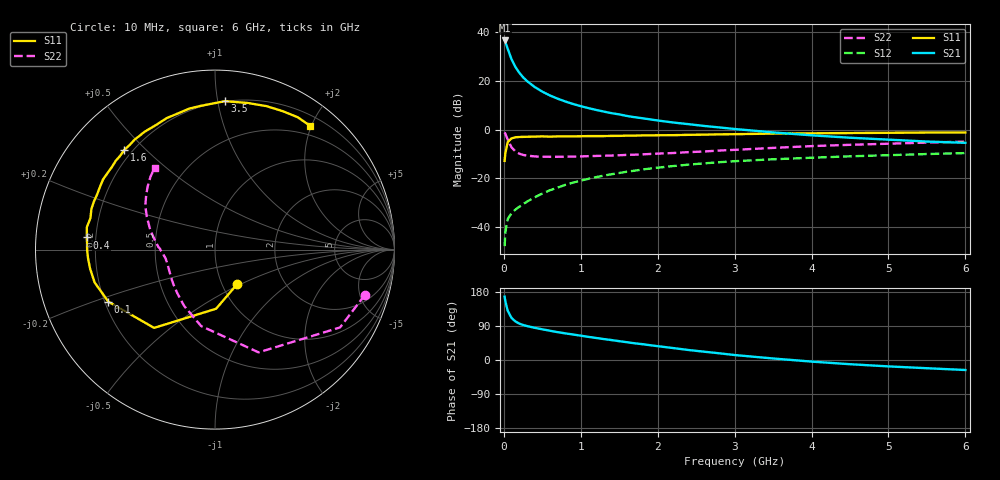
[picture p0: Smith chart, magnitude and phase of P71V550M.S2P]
! SIEMENS Small Signal Semiconductors
! BFP196
! Si NPN RF Bipolar Junction Transistor in SOT143
! VCE = 1.5 V  IC = 50 mA
! Common Emitter S-Parameters:  May  1996
# GHz  S  MA  R  50
!  f  S11  S21  S12  S22
! GHz  MAG  ANG  MAG  ANG  MAG  ANG  MAG  ANG
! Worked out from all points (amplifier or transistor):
!   36 points, 10 MHz to 6 GHz, reference 50 ohm
!   highest |S21| = 36.5 dB at 10 MHz (marker M1)
!   |S21| within 3 dB of that: start of sweep to 45.71 MHz
!   unconditionally stable (mu >= 1): 402.8 MHz to 4.816 GHz
!   at 250 MHz: K = 0.87, MSG = 26.0 dB, |S12| = -30.5 dB
!   at 1.4 GHz: K = 1.09, MAG = 10.6 dB, |S12| = -18.3 dB
!   at 6 GHz: K = 0.99, MSG = 2.1 dB, |S12| = -9.6 dB
!   S11 on the Smith chart (normalised r, x): 10 MHz: 1.17, -0.48; 100 MHz: 0.21, -0.22; 400 MHz: 0.17, +0.05; 1.6 GHz: 0.17, +0.43; 3.5 GHz: 0.20, +1.05; 6 GHz: 0.35, +1.98
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0.01  0.229 -57.8  66.76 167.2  0.0041 79.4  0.8725 -16.8
0.02  0.3295 -88.9  61.61 154.7  0.008 70.0  0.8207 -31.9
0.05  0.5527 -127.9  45.22 130.1  0.0147 53.2  0.622 -67.0
0.1  0.6613 -154.0  27.49 110.9  0.0194 47.9  0.4328 -100.3
0.15  0.6952 -164.7  19.2 101.8  0.023 49.0  0.3576 -118.8
0.2  0.7044 -171.5  14.67 96.2  0.0262 51.7  0.3215 -130.7
0.25  0.7088 -176.0  11.77 92.4  0.0297 54.5  0.3026 -139.7
0.3  0.7123 -179.5  9.865 89.6  0.0334 57.0  0.2932 -145.2
0.4  0.7169 174.6  7.463 85.0  0.0409 60.2  0.2822 -153.6
0.5  0.7251 170.1  5.979 81.0  0.0489 61.7  0.2781 -159.0
0.6  0.7157 165.8  4.982 77.2  0.0573 62.5  0.2771 -162.7
0.7  0.725 161.8  4.285 73.4  0.065 62.7  0.2772 -165.5
0.9  0.7253 154.8  3.339 67.2  0.0819 61.6  0.2793 -169.9
1.1  0.7361 147.9  2.748 61.0  0.0981 59.9  0.2856 -172.9
1.3  0.7362 141.2  2.335 55.2  0.1143 57.3  0.2914 -175.7
1.6  0.7509 132.2  1.9 46.9  0.1371 53.4  0.3033 -179.4
2.2  0.7677 115.5  1.396 31.6  0.1789 44.6  0.3313 173.1
3  0.8041 96.1  1.028 13.1  0.225 32.6  0.3843 161.4
3.5  0.8288 86.2  0.875 4.0  0.2466 25.7  0.4216 154.3
4.5  0.8493 70.2  0.681 -11.1  0.2834 13.6  0.4875 141.9
5.5  0.8695 58.0  0.569 -21.7  0.3155 2.8  0.5418 131.6
6  0.87 52.5  0.535 -26.4  0.3303 -2.9  0.5666 126.5
